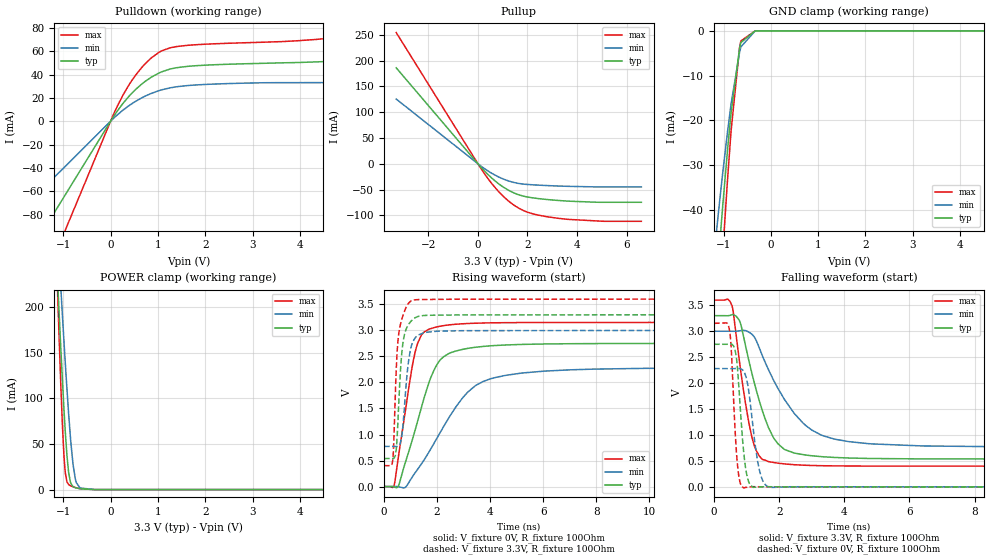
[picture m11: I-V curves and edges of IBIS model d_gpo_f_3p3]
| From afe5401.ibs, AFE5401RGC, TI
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|   d_gpo_f_3p3 Model
[Model]   d_gpo_f_3p3
Model_type   3-state
Polarity   Non-Inverting
Vmeas = 1.65
Vref = 0
Cref = 5pF
Rref = 50
|   typ   min   max
|   (nom PVT)   (fast PVT)   (slow PVT)
C_comp   1.693e-12   1.633e-12   1.756e-12
| Where nom  PVT is Nominal Process, 3.3V, 27C
|   Fast PVT is Strong Process,  3.6V, -40C
|   Slow PVT is Weak Process,   3V, 125C
[Voltage Range]   3.3   3   3.6
|Junction Temperature
[Temperature Range]   27   125   -40
[Pullup Reference]   3.3   3   3.6
[Pulldown Reference]   0   0   0
[Power Clamp Reference]   3.3   3   3.6
[GND Clamp Reference]   0   0   0
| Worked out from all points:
|   slope of the pulldown table from 0 to 0.495 V, typ, clamps not added: 19.1 ohm
|   slope of the pullup table from 0 to 0.495 V, typ, clamps not added: 19.8 ohm
|   POWER clamp passes 1 mA (typ) near -0.65 V on its own axis
|   falling waveform, V_fixture 3.3V, R_fixture 100Ohm: 20-80 % time 756ps typ, 1.29ns min, 463ps max; typ from 3.3 V to 0.539 V
|   rising waveform, V_fixture 0V, R_fixture 100Ohm: 20-80 % time 993ps typ, 1.74ns min, 588ps max; typ from 0 V to 2.75 V
|   rising waveform, V_fixture 3.3V, R_fixture 100Ohm: 20-80 % time 201ps typ, 250ps min, 182ps max; typ from 0.539 V to 3.3 V
|   falling waveform, V_fixture 0V, R_fixture 100Ohm: 20-80 % time 201ps typ, 280ps min, 153ps max; typ from 2.75 V to 0 V
[Pulldown]
|   Voltage   I(typ)   I(min)   I(max)
-3.3V     -217.4mA   -133.2mA   -321.9mA
-3mV      -197.6uA   -121.1uA   -292.6uA
257.4mV   15.06mA    9.341mA    22.04mA
534mV     27.43mA    17.19mA    39.76mA
696mV     33.08mA    20.83mA    47.74mA
855mV     37.6mA     23.77mA    54.06mA
1.079V    42.35mA    26.9mA     60.33mA
1.254V    44.71mA    28.6mA     62.89mA
1.61V     46.97mA    30.51mA    65.02mA
2.679V    49.08mA    32.49mA    67.08mA
4.505V    51.1mA     33.09mA    70.61mA
6.6V      54.03mA    33.13mA    80.49mA
[GND Clamp]
|   Voltage   I(typ)   I(min)   I(max)
-3.3V     -1.237A    -1.056A    -1.383A
-1.185V   -62.02mA   -48.47mA   -79.23mA
-1.09V    -48.68mA   -38.74mA   -62.09mA
-1.016V   -38.95mA   -31.63mA   -49.47mA
-914.1mV  -26.39mA   -22.38mA   -33mA
-840mV    -18.26mA   -16.29mA   -22.27mA
-660mV    -3.853mA   -4.762mA   -3.675mA
-632.4mV  -2.604mA   -3.574mA   -2.256mA
-330mV    -1.092uA   -13.07uA   -101.3nA
6.6V      0A         0A         0A
[Pullup]
|   Voltage   I(typ)   I(min)   I(max)
-3.3V     186.2mA    125.6mA    254.7mA
192mV     -10.4mA    -6.983mA   -14.27mA
513mV     -25.83mA   -17.2mA    -35.64mA
800.4mV   -37.54mA   -24.78mA   -52.15mA
1.311V    -53.36mA   -34.52mA   -75.28mA
1.628V    -59.93mA   -38.12mA   -85.64mA
1.935V    -63.95mA   -39.94mA   -92.76mA
2.231V    -66.33mA   -40.93mA   -97.34mA
2.835V    -69.65mA   -42.45mA   -103.2mA
3.633V    -72.58mA   -43.82mA   -107.9mA
4.963V    -74.81mA   -44.9mA    -111.4mA
6.6V      -74.81mA   -44.9mA    -111.7mA
[POWER Clamp]
|   Voltage   I(typ)   I(min)   I(max)
-3.3V     2.973A     2.513A     4.173A
-1.115V   224.2mA    279.7mA    208.8mA
-1.089V   194.8mA    255.2mA    168mA
-1.053V   155.8mA    222.2mA    115.5mA
-1.018V   119.2mA    190.5mA    69.8mA
-984mV    86.76mA    161.1mA    35.87mA
-956.4mV  62.6mA     137.8mA    18.2mA
-921mV    36.52mA    109mA      8.361mA
-841.5mV  6.984mA    52.62mA    4.074mA
-747mV    2.117mA    12.15mA    2.312mA
-645mV    931.7uA    1.77mA     936.9uA
6.6V      0A         0A         0A
[Ramp]
R_load = 100
|   typ   min   max
dV/dt_r   1.64937/9.92767e-10   1.3677/1.73809e-09   1.89157/5.87245e-10
dV/dt_f   1.65672/7.51702e-10   1.33737/1.29106e-09   1.91895/4.62062e-10
[Falling Waveform]
V_fixture = 3.3V
V_fixture_min = 3V
V_fixture_max = 3.6V
R_fixture = 100Ohm
|   Time   V(typ)   V(min)   V(max)
0s        3.3V       3V         3.6V
545ps     3.317V     2.999V     3.502V
800ps     3.174V     3.01V      2.32V
1.16ns    2.193V     2.943V     966.2mV
1.39ns    1.658V     2.678V     596.4mV
1.67ns    1.147V     2.26V      488.8mV
2.145ns   731.1mV    1.703V     446mV
2.725ns   624.3mV    1.235V     420.7mV
3.705ns   568.9mV    921.3mV    406.8mV
14.99ns   538.8mV    771mV      401.8mV
[Rising Waveform]
V_fixture = 0V
V_fixture_min = 0V
V_fixture_max = 0V
R_fixture = 100Ohm
|   Time   V(typ)   V(min)   V(max)
0s        1.162nV    64.92nV    547pV
385ps     -7.748mV   540.8uV    26.76mV
570ps     41.9mV     -5.871mV   661.1mV
1.165ns   1.067V     258.1mV    2.561V
1.41ns    1.517V     433.2mV    2.907V
1.715ns   2.025V     679.4mV    3.026V
2.435ns   2.553V     1.313V     3.104V
3.18ns    2.656V     1.824V     3.132V
4.215ns   2.71V      2.097V     3.146V
14.99ns   2.749V     2.279V     3.153V
[Rising Waveform]
V_fixture = 3.3V
V_fixture_min = 3V
V_fixture_max = 3.6V
R_fixture = 100Ohm
|   Time   V(typ)   V(min)   V(max)
0s        538.8mV    771mV      401.8mV
330ps     537.8mV    771.1mV    500.1mV
465ps     720.7mV    768.4mV    2.271V
530ps     1.285V     773.9mV    2.81V
620ps     2.206V     840.7mV    3.114V
770ps     2.914V     1.515V     3.361V
910ps     3.101V     2.341V     3.51V
1.07ns    3.202V     2.757V     3.576V
2.015ns   3.292V     2.984V     3.596V
14.99ns   3.3V       3V         3.6V
[Falling Waveform]
V_fixture = 0V
V_fixture_min = 0V
V_fixture_max = 0V
R_fixture = 100Ohm
|   Time   V(typ)   V(min)   V(max)
0s        2.749V     2.28V      3.153V
470ps     2.752V     2.28V      3.033V
530ps     2.753V     2.28V      2.629V
640ps     2.643V     2.281V     1.158V
715ps     2.315V     2.283V     451.8mV
905ps     701.3mV    2.231V     -15.11mV
1.075ns   79.48mV    1.799V     1.737mV
1.385ns   144.7uV    341.1mV    4.736mV
1.705ns   5.173mV    -10.28mV   2.361mV
14.99ns   13.17nV    742.6nV    1.363nV
